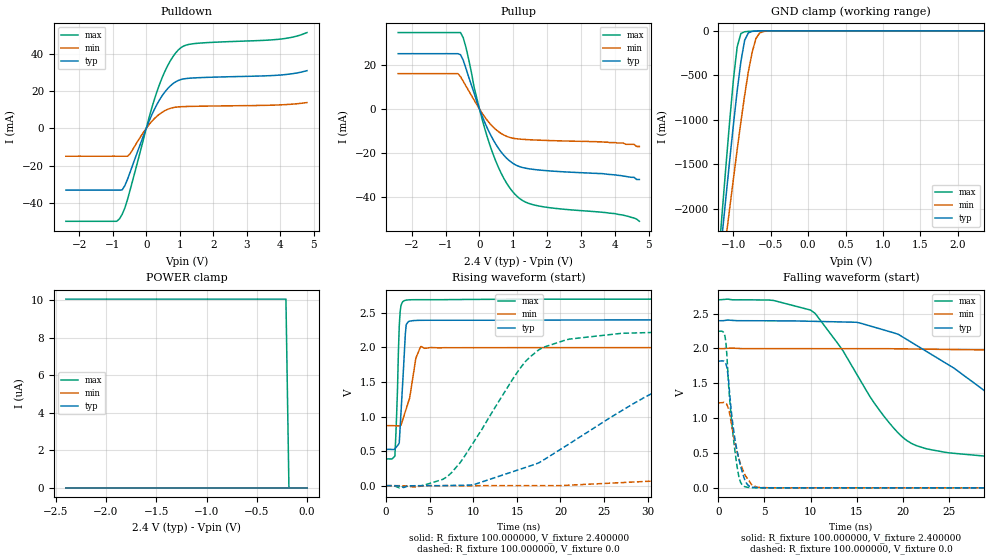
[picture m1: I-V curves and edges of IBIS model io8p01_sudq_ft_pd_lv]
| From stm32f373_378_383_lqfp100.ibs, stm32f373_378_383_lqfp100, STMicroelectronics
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|   Model io8p01_sudq_ft_pd_lv
[Model]  io8p01_sudq_ft_pd_lv
Model_type I/O
Polarity   Non-Inverting
Enable   Active-Low
Vinl =   0.720000V
Vinh =   1.680000V
Vmeas =  1.200000V
Cref =   50.000000pF
Rref =   100.000000M
Vref =   0.0V
C_comp   1.970100pF   1.887900pF   2.069400pF
[Temperature Range]   25.000000   0.125000k   -40.000000
[Pullup Reference]   2.400000V   2.000000V   2.700000V
[Pulldown Reference]   0.0V   0.0V   0.0V
[POWER Clamp Reference]   2.400000V   2.000000V   2.700000V
[GND Clamp Reference]   0.0V   0.0V   0.0V
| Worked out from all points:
|   slope of the pulldown table from 0 to 0.36 V, typ, clamps not added: 25.5 ohm
|   slope of the pullup table from 0 to 0.36 V, typ, clamps not added: 28.4 ohm
|   GND clamp passes 1 mA (typ) near -0.64 V on its own axis
|   rising waveform, R_fixture 100.000000, V_fixture 2.400000: 20-80 % time 499ps typ, 1.06ns min, 336ps max; typ from 0.525 V to 2.4 V
|   rising waveform, R_fixture 100.000000, V_fixture 0.0: 20-80 % time 14.6ns typ, 43.7ns min, 6.88ns max; typ from 0 V to 1.82 V
|   falling waveform, R_fixture 100.000000, V_fixture 2.400000: 20-80 % time 12.9ns typ, 32.5ns min, 7.07ns max; typ from 2.4 V to 0.525 V
|   falling waveform, R_fixture 100.000000, V_fixture 0.0: 20-80 % time 1.15ns typ, 1.36ns min, 910ps max; typ from 1.82 V to 0 V
[Pulldown]
|Voltage   I(typ)   I(min)   I(max)
-2.4V     -33.16mA   -14.98mA   -49.86mA
-880mV    -33.16mA   -14.98mA   -49.86mA
-800mV    -33.16mA   -14.98mA   -48.55mA
-640mV    -30.75mA   -14.98mA   -42.76mA
-480mV    -23.43mA   -13.57mA   -32.92mA
80mV      3.651mA    1.905mA    5.506mA
400mV     15.37mA    7.665mA    23.73mA
720mV     22.75mA    10.69mA    36.23mA
1.04V     26.18mA    11.57mA    43.27mA
1.52V     27.09mA    11.81mA    45.55mA
4V        28.55mA    12.55mA    47.81mA
4.8V      30.9mA     13.81mA    51.31mA
[Pullup]
|Voltage   I(typ)   I(min)   I(max)
-2.4V     25.2mA     16.13mA    34.79mA
-640mV    25.2mA     16.13mA    34.79mA
-560mV    24.71mA    14.75mA    34.79mA
-400mV    18.51mA    10.48mA    28.09mA
-160mV    7.338mA    4.152mA    10.02mA
80mV      -3.229mA   -1.94mA    -4.736mA
400mV     -13.82mA   -8.081mA   -20.45mA
800mV     -22.31mA   -12.38mA   -33.66mA
1.2V      -26.24mA   -13.65mA   -40.83mA
1.76V     -27.69mA   -14.12mA   -44.07mA
4V        -29.9mA    -15.2mA    -47.5mA
4.72V     -32mA      -17mA      -51mA
[GND_clamp]
|Voltage   I(typ)   I(min)   I(max)
-2.4V     -9.788A    -9.782A    -9.734A
-1.2V     -2.718A    -3.021A    -2.568A
-1.15V    -2.29A     -2.675A    -2.036A
-1.1V     -1.868A    -2.333A    -1.515A
-1.05V    -1.454A    -1.995A    -1.012A
-950mV    -674.5mA   -1.337A    -180.6mA
-900mV    -345.2mA   -1.023A    -29.74mA
-850mV    -106.4mA   -726mA     -10.14mA
-750mV    -6.411mA   -244mA     -4.042mA
-700mV    -2.572mA   -88.62mA   -2.346mA
-600mV    -429.6uA   -7.75mA    -383.5uA
2.35V     59.77uA    46.33uA    66.89uA
[POWER_clamp]
|Voltage   I(typ)   I(min)   I(max)
-2.4V     0A         0A         10.06uA
-210mV    0A         0A         10.06uA
-180mV    0A         0A         0A
0V        0A         0A         0A
[Ramp]
| variable   typ   min   max
dV/dt_r  1.09218/14.55718n   0.73266/43.64565n   1.34874/6.87247n
dV/dt_f  1.12429/12.86053n   0.67801/32.45722n   1.38701/7.06387n
R_load = 100.000000
[Rising Waveform]
R_fixture= 100.000000
V_fixture= 2.400000
V_fixture_min= 2.000000
V_fixture_max= 2.700000
|time   V(typ)   V(min)   V(max)
0s        524.8mV    868.7mV    387.2mV
1.001ns   533mV      867mV      427.7mV
1.301ns   579.7mV    865.4mV    1.395V
1.502ns   618.4mV    864.7mV    2.307V
1.602ns   837.8mV    864.4mV    2.512V
2.102ns   1.961V     1.034V     2.677V
2.302ns   2.331V     1.113V     2.684V
3.403ns   2.39V      1.843V     2.691V
4.004ns   2.392V     2.014V     2.691V
49.85ns   2.399V     1.999V     2.699V
[Rising Waveform]
R_fixture= 100.000000
V_fixture= 0.0
V_fixture_min= 0.0
V_fixture_max= 0.0
|time   V(typ)   V(min)   V(max)
0s        1.768nV    15.89nV    1.355nV
7.007ns   1.867mV    822uV      130.1mV
15.02ns   222.8mV    610.6uV    1.635V
17.52ns   330.7mV    351.7uV    1.966V
27.03ns   1.085V     44.44mV    2.204V
34.53ns   1.55V      90.81mV    2.229V
43.04ns   1.723V     239mV      2.246V
84.08ns   1.82V      945.5mV    2.248V
103.1ns   1.82V      1.111V     2.248V
249.2ns   1.82V      1.221V     2.248V
[Falling Waveform]
R_fixture= 100.000000
V_fixture= 2.400000
V_fixture_min= 2.000000
V_fixture_max= 2.700000
|time   V(typ)   V(min)   V(max)
0s        2.399V     1.999V     2.699V
10.01ns   2.391V     1.998V     2.551V
15.02ns   2.376V     1.997V     1.633V
20.02ns   2.165V     1.994V     725.2mV
29.53ns   1.332V     1.979V     449.6mV
35.04ns   877.6mV    1.964V     425.1mV
42.54ns   673.2mV    1.851V     405.8mV
67.07ns   552.7mV    1.286V     389.2mV
85.59ns   536.1mV    1.035V     387.2mV
249.2ns   524.8mV    868.7mV    387.2mV
[Falling Waveform]
R_fixture= 100.000000
V_fixture= 0.0
V_fixture_min= 0.0
V_fixture_max= 0.0
|time   V(typ)   V(min)   V(max)
0s        1.82V      1.221V     2.248V
700.7ps   1.801V     1.221V     2.178V
800.8ps   1.783V     1.214V     2.095V
1.001ns   1.652V     1.164V     1.701V
1.401ns   1.088V     921.6mV    989mV
1.802ns   687.3mV    646.2mV    513.2mV
2.302ns   364.2mV    381.5mV    115.5mV
2.903ns   104.2mV    178.7mV    14.94mV
4.705ns   1.559mV    3.204mV    789.6uV
49.85ns   1.768nV    15.89nV    1.355nV
